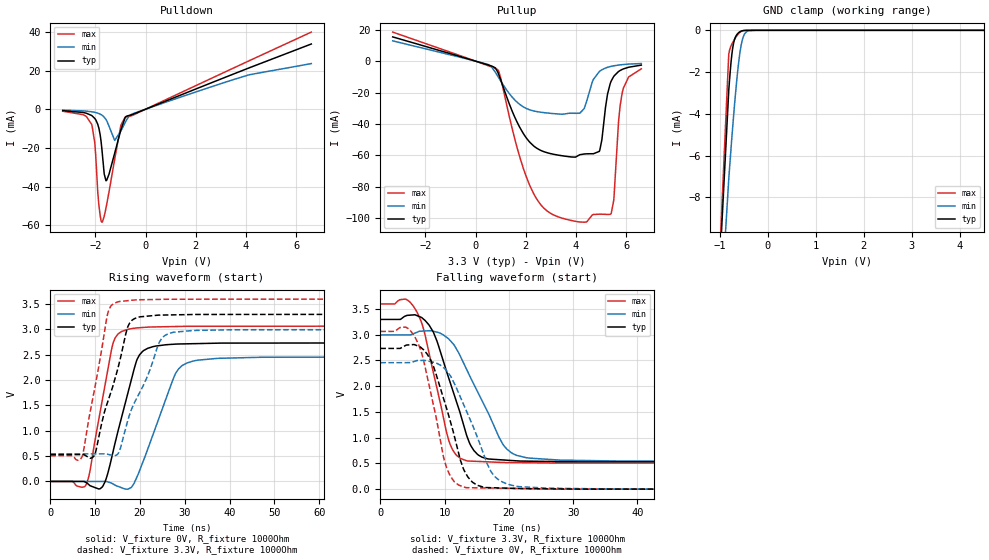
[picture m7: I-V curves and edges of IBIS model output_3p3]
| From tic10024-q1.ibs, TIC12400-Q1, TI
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|   output_3p3 Model
[Model]   output_3p3
Model_type   3-state
Polarity   Non-Inverting
Vmeas = 1.65
Vref = 0
Cref = 2pF
Rref = 100000
|   typ   min   max
C_comp   1.96626E-12F   1.82658E-12F   2.04005E-12F
| Where nom  PVT is Nominal Process, 3.3V, 27C
|   Fast PVT is Strong Process,  3.6V, -40C
|   Slow PVT is Weak Process,   3.0V, 150C
[Voltage Range]   3.3   3   3.6
|Junction Temperature
[Temperature Range]   27   150   -40
[Pullup Reference]   3.3   3   3.6
[Pulldown Reference]   0   0   0
[Power Clamp Reference]   3.3   3   3.6
[GND Clamp Reference]   0   0   0
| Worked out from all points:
|   slope of the pulldown table from 0 to 0.495 V, typ, clamps not added: 191 ohm
|   slope of the pullup table from 0 to 0.495 V, typ, clamps not added: 206 ohm
|   GND clamp passes 1 mA (typ) near -0.74 V on its own axis
|   falling waveform, V_fixture 3.3V, R_fixture 1000Ohm: 20-80 % time 4.18ns typ, 5.63ns min, 3.27ns max; typ from 3.29 V to 0.528 V
|   rising waveform, V_fixture 0V, R_fixture 1000Ohm: 20-80 % time 4.72ns typ, 6.04ns min, 3.74ns max; typ from 0 V to 2.73 V
|   rising waveform, V_fixture 3.3V, R_fixture 1000Ohm: 20-80 % time 5.11ns typ, 6.59ns min, 3.75ns max; typ from 0.528 V to 3.29 V
|   falling waveform, V_fixture 0V, R_fixture 1000Ohm: 20-80 % time 3.71ns typ, 4.79ns min, 3.03ns max; typ from 2.73 V to 0 V
[Pulldown]
|   Voltage   I(typ)   I(min)   I(max)
-3.3V     -747uA     -467.9uA   -1.035mA
-2.152V   -3.227mA   -1.312mA   -7.724mA
-2.023V   -4.768mA   -1.616mA   -17.35mA
-1.865V   -9.563mA   -2.221mA   -49mA
-1.736V   -21.17mA   -3.092mA   -58.41mA
-1.647V   -33.54mA   -4.102mA   -55.3mA
-1.548V   -36.69mA   -5.964mA   -49.19mA
-1.231V   -22.77mA   -16.1mA    -25.9mA
-983.4mV  -10.63mA   -11.28mA   -8.279mA
-815.1mV  -4.378mA   -6.911mA   -4.048mA
3.422V    17.79mA    14.98mA    20.8mA
6.6V      33.72mA    23.58mA    39.87mA
[GND Clamp]
|   Voltage   I(typ)   I(min)   I(max)
-3.3V     -1.398A    -1.627A    -1.283A
-1.201V   -20.14mA   -21.7mA    -20.85mA
-815.1mV  -2.889mA   -7.139mA   -1.145mA
-765.6mV  -1.488mA   -5.607mA   -732uA
-716.1mV  -636.6uA   -4.163mA   -511.7uA
-676.5mV  -328.4uA   -3.095mA   -363uA
-627mV    -152.5uA   -1.921mA   -203.1uA
-557.7mV  -39.62uA   -728.9uA   -54.52uA
-518.1mV  -14.44uA   -344.2uA   -18.42uA
-438.9mV  -1.245uA   -54.77uA   -1.199uA
-260.7mV  0A         -456.6nA   0A
6.6V      0A         0A         0A
[Pullup]
|   Voltage   I(typ)   I(min)   I(max)
-3.3V     15.5mA     12.97mA    18.57mA
887.7mV   -7.076mA   -9.679mA   -5.491mA
1.729V    -41.28mA   -27.17mA   -59.44mA
2.323V    -54.17mA   -31.75mA   -84.75mA
2.967V    -58.85mA   -33.21mA   -96.81mA
4.115V    -59.95mA   -33.19mA   -102.5mA
4.927V    -57.51mA   -6.588mA   -97.54mA
5.402V    -12.6mA    -3.268mA   -97.1mA
5.501V    -9.701mA   -2.944mA   -88.72mA
5.689V    -6.623mA   -2.471mA   -39.58mA
5.838V    -5.254mA   -2.191mA   -20.3mA
6.6V      -2.495mA   -1.482mA   -4.859mA
[POWER Clamp]
|   Voltage   I(typ)   I(min)   I(max)
-3.3V     0A         0A         0A
0V        0A         0A         0A
6.6V      0A         0A         0A
[Ramp]
R_load = 1000
|   typ   min   max
dV/dt_r   1.63914/4.72145e-09   1.47324/6.03762e-09   1.83738/3.74142e-09
dV/dt_f   1.65964/4.17369e-09   1.47028/5.6258e-09   1.85278/3.26958e-09
[Falling Waveform]
V_fixture = 3.3V
V_fixture_min = 3V
V_fixture_max = 3.6V
R_fixture = 1000Ohm
C_fixture = 0F
|   Time   V(typ)   V(min)   V(max)
0s        3.294V     2.993V     3.595V
4.702ns   3.378V     2.994V     3.621V
6.344ns   3.336V     3.067V     3.26V
7.56ns    3.189V     3.075V     2.656V
10.77ns   2.11V      2.899V     902.5mV
13.44ns   1.04V      2.321V     550.5mV
15.27ns   660.5mV    1.855V     538mV
19.03ns   567.5mV    879.1mV    518mV
22.67ns   544.1mV    611.7mV    512.7mV
100ns     528.3mV    543mV      506.6mV
[Rising Waveform]
V_fixture = 0V
V_fixture_min = 0V
V_fixture_max = 0V
R_fixture = 1000Ohm
C_fixture = 0F
|   Time   V(typ)   V(min)   V(max)
0s        -50.86uV   37.86uV    -35.52uV
7.984ns   -22.34mV   -167.3uV   -65.14mV
12.25ns   -793.4uV   -276.8uV   1.915V
14.08ns   615.4mV    -54.16mV   2.745V
17ns      1.635V     -152.4mV   2.991V
19.2ns    2.366V     61.73mV    3.025V
20.59ns   2.563V     365.4mV    3.034V
27.8ns    2.706V     2.101V     3.053V
30.52ns   2.712V     2.336V     3.058V
100ns     2.732V     2.455V     3.062V
[Rising Waveform]
V_fixture = 3.3V
V_fixture_min = 3V
V_fixture_max = 3.6V
R_fixture = 1000Ohm
C_fixture = 0F
|   Time   V(typ)   V(min)   V(max)
0s        528.3mV    543mV      506.6mV
7.078ns   528.6mV    543.2mV    483.4mV
9.895ns   525.2mV    543.3mV    1.826V
12.73ns   1.549V     536.7mV    3.279V
15.03ns   2.214V     536.9mV    3.538V
17.18ns   3.018V     1.167V     3.562V
18.2ns    3.174V     1.44V      3.571V
24.31ns   3.278V     2.74V      3.588V
26.32ns   3.281V     2.911V     3.591V
100ns     3.294V     2.993V     3.595V
[Falling Waveform]
|Gnd
V_fixture = 0V
V_fixture_min = 0V
V_fixture_max = 0V
R_fixture = 1000Ohm
C_fixture = 0F
|   Time   V(typ)   V(min)   V(max)
0s        2.732V     2.455V     3.062V
4.641ns   2.802V     2.455V     3.082V
6.233ns   2.759V     2.498V     2.718V
7.26ns    2.627V     2.491V     2.206V
10.26ns   1.589V     2.308V     438.6mV
11.47ns   1.052V     2.061V     150.6mV
13.25ns   316.8mV    1.559V     31.43mV
17.33ns   28.06mV    320.6mV    21.12mV
21.26ns   14.43mV    54.52mV    13.24mV
100ns     -50.89uV   37.87uV    -35.5uV
